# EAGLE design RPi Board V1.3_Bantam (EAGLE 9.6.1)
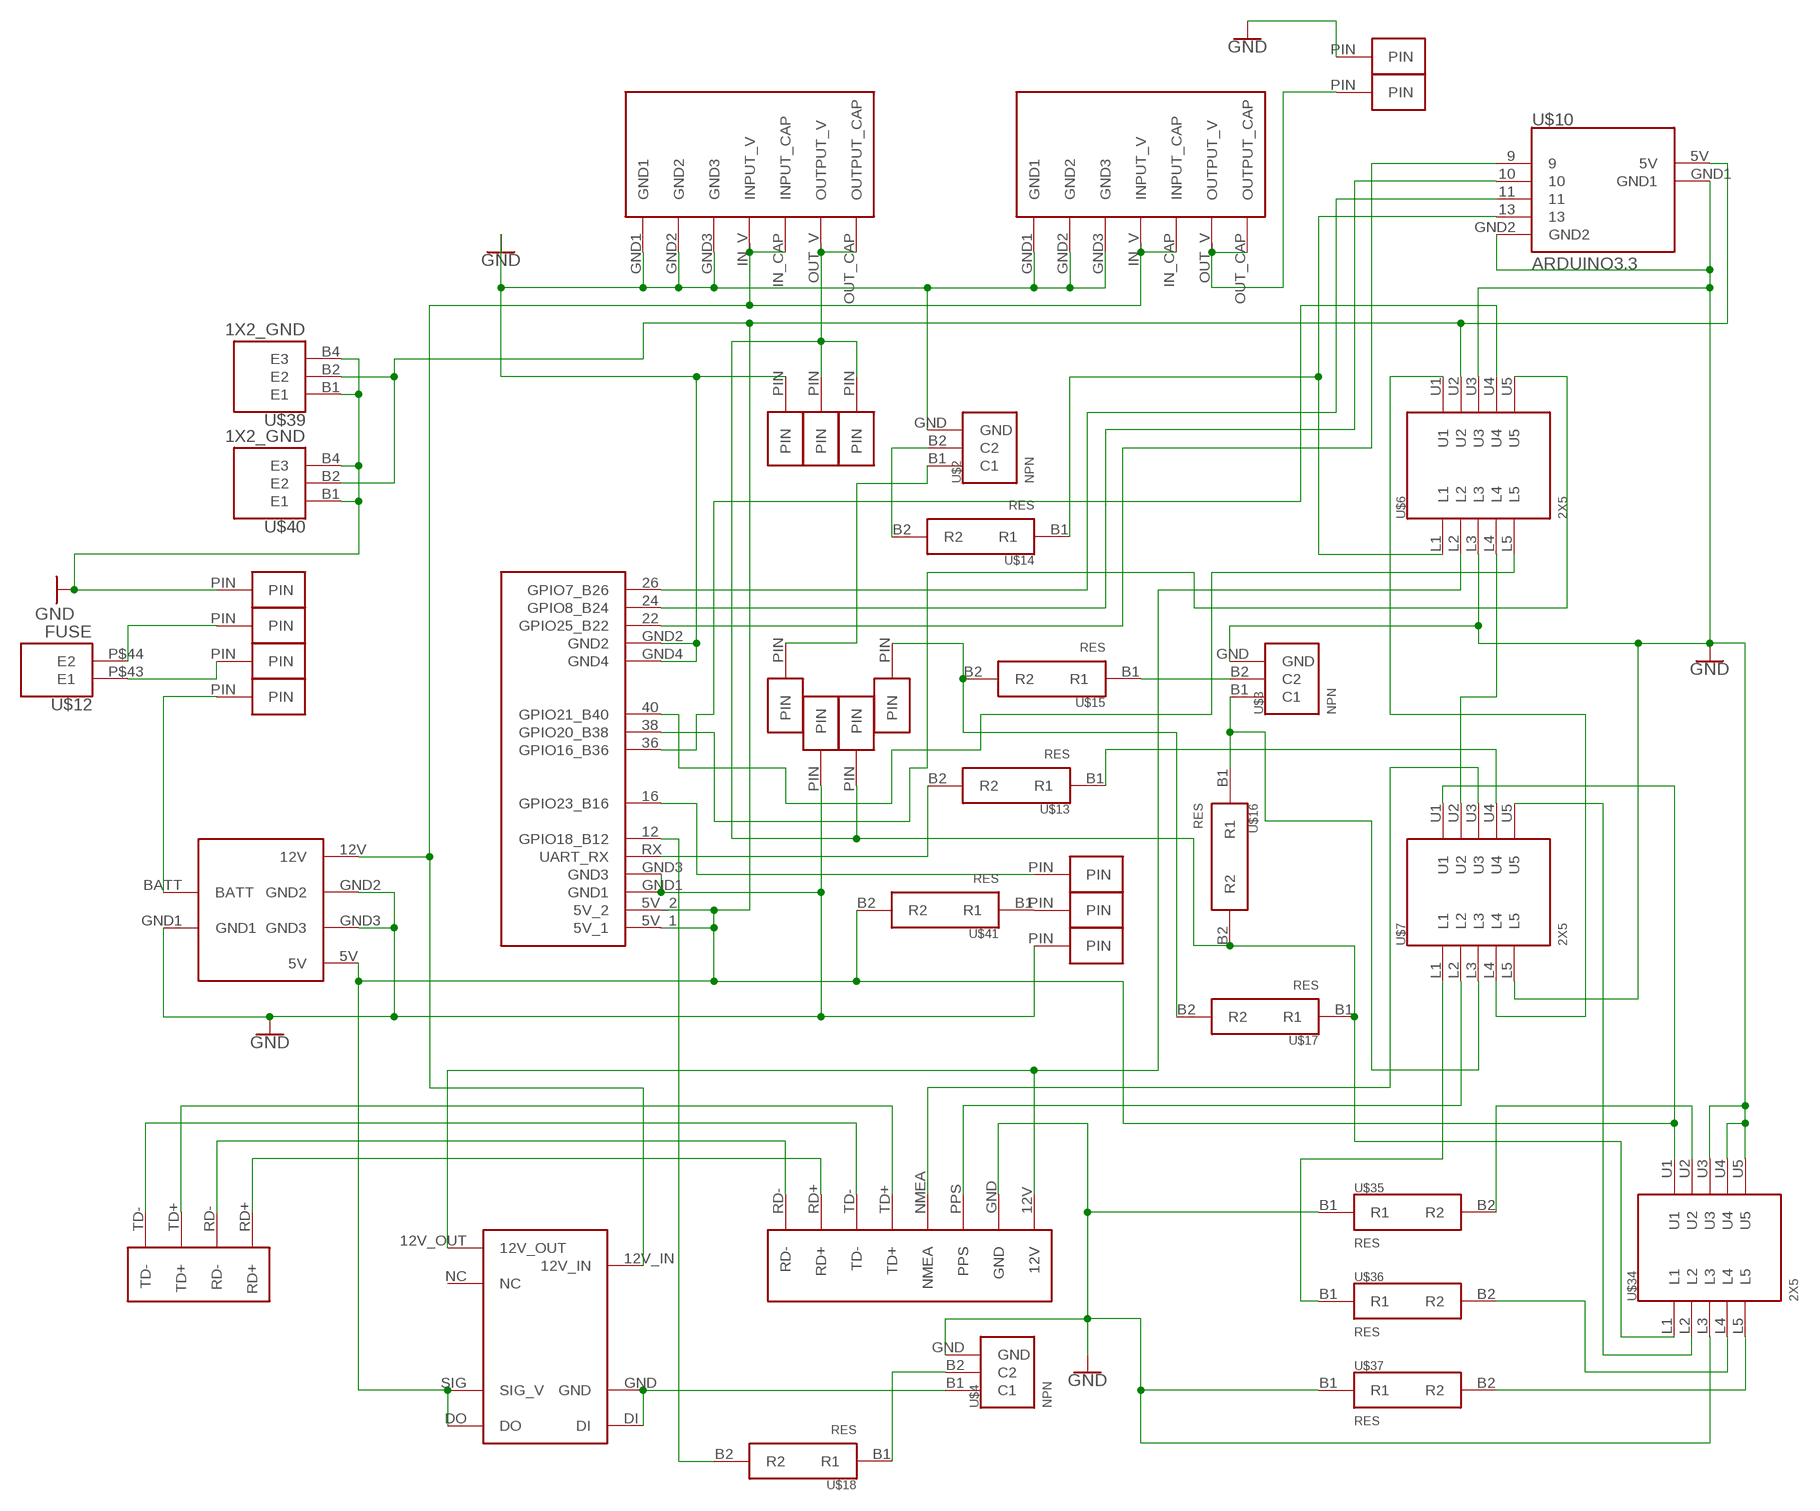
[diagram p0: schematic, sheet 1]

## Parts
U$1  RPI_1X20  [F_RPI_1X20]
U$2  NPN  [F_NPN]
U$3  NPN  [F_NPN]
U$4  NPN  [F_NPN]
U$5  LIDAR  [F_LIDAR]
U$6  2X5  [F_2X5]
U$7  2X5  [F_2X5]
U$8  3.3V_REG  [F_3.3V_REG]
U$9  9V_REG  [F_9V_REG]
U$10  ARDUINO3.3  [F_ARDUINO3.3]
U$11  ETH  [F_ETH]
U$12  FUSE  [F_FUSE]
U$13  RES  [F_RES]
U$14  RES  [F_RES]
U$15  RES  [F_RES]
U$16  RES  [F_RES]
U$17  RES  [F_RES]
U$18  RES  [F_RES]
U$19  1X1  [F_1X1]
U$20  1X1  [F_1X1]
U$21  1X1  [F_1X1]
U$22  1X1  [F_1X1]
U$23  12V_5V_REG  [F_12V_5V_REG]
U$24  1X1  [F_1X1]
U$25  RELAY  [F_RELAY]
U$26  1X1  [F_1X1]
U$27  1X1  [F_1X1]
U$28  1X1  [F_1X1]
U$29  1X1  [F_1X1]
U$30  1X1  [F_1X1]
U$31  1X1  [F_1X1]
U$32  1X1  [F_1X1]
U$33  1X1  [F_1X1]
U$34  2X5  [F_2X5]
U$35  RES  [F_RES]
U$36  RES  [F_RES]
U$37  RES  [F_RES]
U$38  1X1  [F_1X1]
U$39  1X2_GND  [F_1X2_GND]
U$40  1X2_GND  [F_1X2_GND]
U$41  RES  [F_RES]
U$42  1X1  [F_1X1]
U$43  1X1  [F_1X1]

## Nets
GND: U$1.GND1 U$1.GND2 U$1.GND3 U$1.GND4 U$2.GND U$3.GND U$4.GND U$5.GND U$6.L3 U$6.U3 U$7.L5 U$8.GND1 U$8.GND2 U$8.GND3 U$9.GND1 U$9.GND2 U$9.GND3 U$10.GND1 U$10.GND2 U$22.PIN U$23.GND1 U$23.GND2 U$23.GND3 U$26.PIN U$28.PIN U$30.PIN U$34.L3 U$34.U3 U$34.U4 U$34.U5 U$35.B1(R1) U$37.B1(R1) U$39.B1(E1) U$39.B4(E3) U$40.B1(E1) U$40.B4(E3) U$43.PIN
N$1: U$12.P$44(E2) U$19.PIN
N$2: U$12.P$43(E1) U$20.PIN
N$3: U$21.PIN U$23.BATT
N$4: U$5.RD- U$11.RD-
N$5: U$5.RD+ U$11.RD+
N$6: U$5.TD- U$11.TD-
N$7: U$41.B1(R1) U$42.PIN
N$8: U$8.OUT_CAP(OUTPUT_CAP) U$8.OUT_V(OUTPUT_V) U$16.B2(R2) U$17.B1(R1) U$24.PIN U$27.PIN U$32.PIN U$34.L1
N$9: U$5.TD+ U$11.TD+
N$10: U$5.PPS U$7.L2
N$11: U$7.U4 U$13.B1(R1)
N$12: U$1.RX(UART_RX) U$13.B2(R2)
N$13: U$5.12V U$6.L2 U$25.12V_OUT
N$14: U$6.U1 U$7.L4
N$15: U$6.L4 U$7.U2
N$16: U$1.5V_1 U$1.5V_2 U$6.U2 U$7.U1 U$10.5V U$23.5V U$25.DO U$25.SIG(SIG_V) U$34.U1 U$39.B2(E2) U$40.B2(E2) U$41.B2(R2)
N$17: U$5.NMEA U$7.U3
N$19: U$1.22(GPIO25_B22) U$10.9
N$20: U$1.24(GPIO8_B24) U$10.10
N$21: U$8.IN_CAP(INPUT_CAP) U$8.IN_V(INPUT_V) U$9.IN_CAP(INPUT_CAP) U$9.IN_V(INPUT_V) U$23.12V U$25.12V_IN
N$22: U$1.26(GPIO7_B26) U$10.11
N$23: U$9.OUT_CAP(OUTPUT_CAP) U$9.OUT_V(OUTPUT_V) U$29.PIN
N$24: U$2.B2(C2) U$14.B2(R2)
N$25: U$6.L1 U$10.13 U$14.B1(R1)
N$26: U$2.B1(C1) U$31.PIN
N$27: U$15.B2(R2) U$17.B2(R2) U$33.PIN
N$28: U$3.B2(C2) U$15.B1(R1)
N$29: U$3.B1(C1) U$7.L3 U$16.B1(R1)
N$30: U$4.B1(C1) U$25.DI U$25.GND
N$31: U$4.B2(C2) U$18.B1(R1)
N$32: U$1.38(GPIO20_B38) U$6.U5
N$33: U$1.12(GPIO18_B12) U$18.B2(R2)
N$34: U$1.36(GPIO16_B36) U$6.U4
N$35: U$7.U5 U$34.L2
N$36: U$34.U2 U$35.B2(R2)
N$37: U$1.16(GPIO23_B16) U$38.PIN
N$38: U$34.L5 U$37.B2(R2)
N$39: U$34.L4 U$36.B2(R2)
N$40: U$7.L1 U$36.B1(R1)
N$42: U$1.40(GPIO21_B40) U$6.L5
Unconnected: U$25.NC

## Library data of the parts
U$1 = OpenMMS_Bantam:RPI_1X20
U$2-U$4 = OpenMMS_Bantam:NPN
U$5 = OpenMMS_Bantam:LIDAR
U$6 U$7 U$34 = OpenMMS_Bantam:2X5
U$8 = OpenMMS_Bantam:3.3V_REG
U$9 = OpenMMS_Bantam:9V_REG
U$10 = OpenMMS_Bantam:ARDUINO3.3
U$11 = OpenMMS_Bantam:ETH
U$12 = OpenMMS_Bantam:FUSE
U$13-U$18 U$35-U$37 U$41 = OpenMMS_Bantam:RES
U$19-U$22 U$24 U$26-U$33 U$38 U$42 U$43 = OpenMMS_Bantam:1X1
U$23 = OpenMMS_Bantam:12V_5V_REG
U$25 = OpenMMS_Bantam:RELAY
U$39 U$40 = OpenMMS_Bantam:1X2_GND

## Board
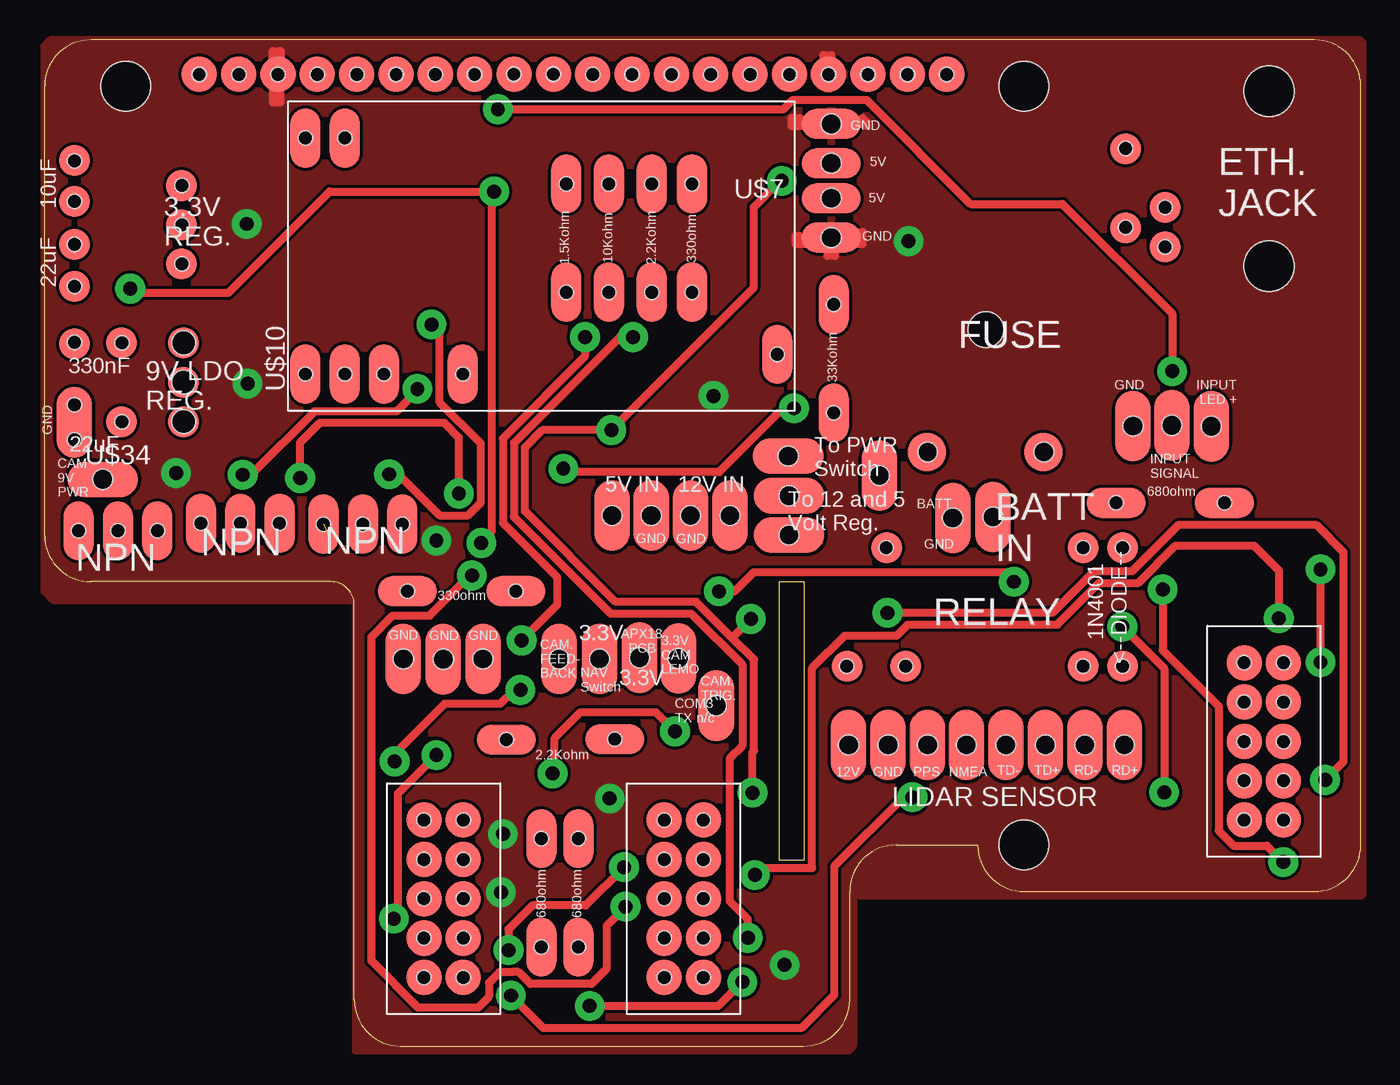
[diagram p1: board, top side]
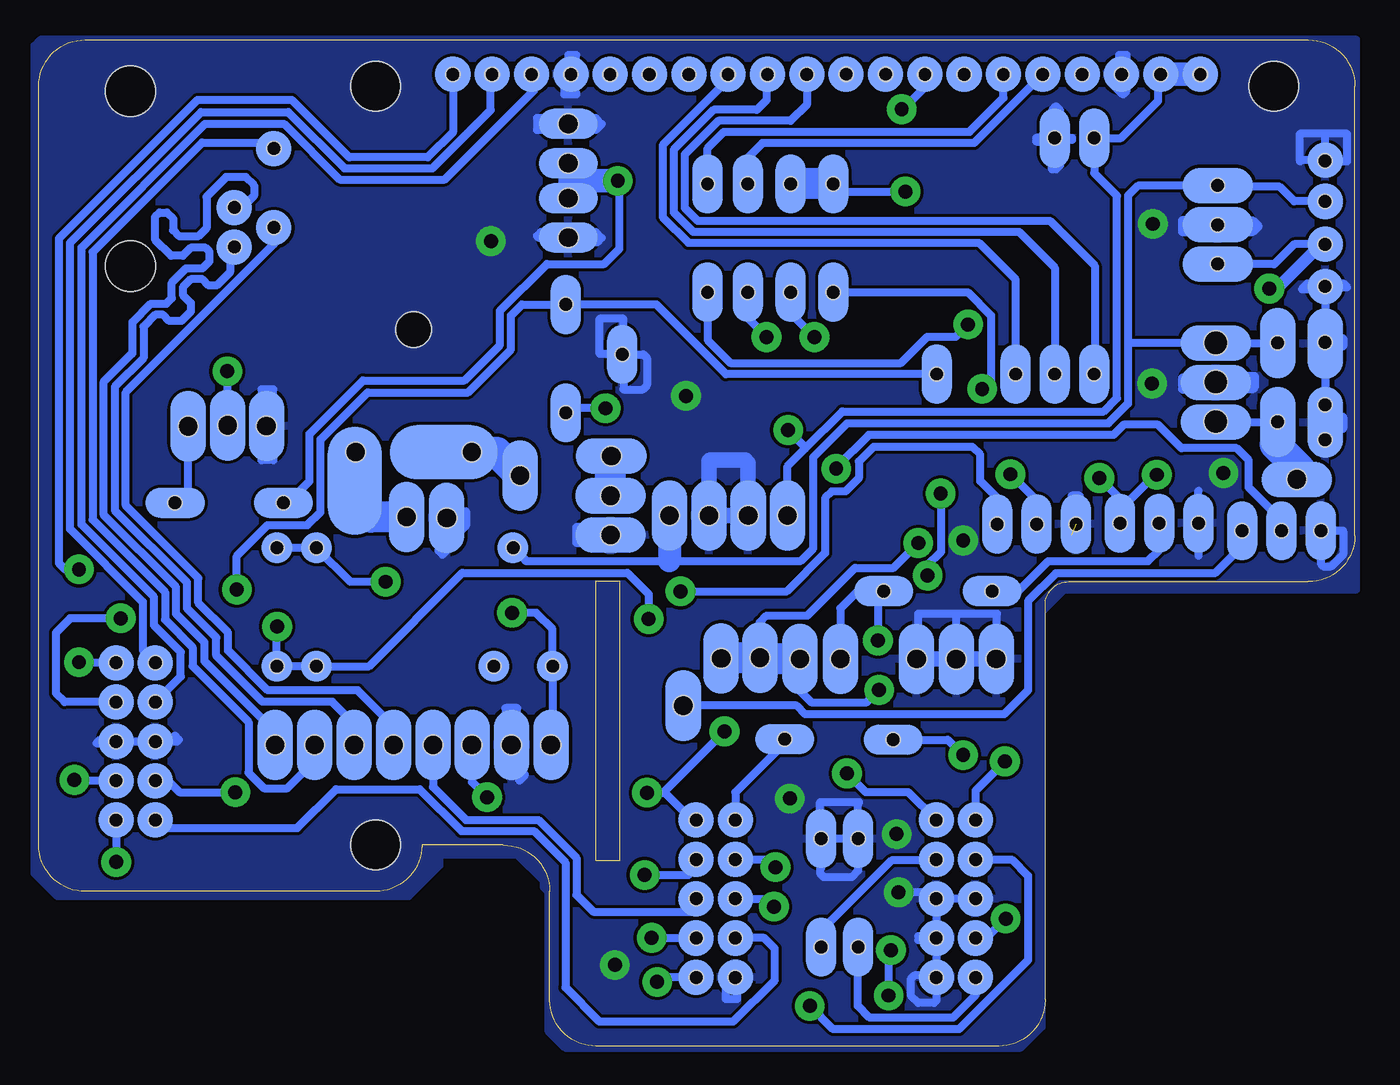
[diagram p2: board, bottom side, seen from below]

Size 85 x 65 mm. Coordinates in mm from the lower left corner, seen from the top.
Outline: 49.05,12 47.45,12 47.45,30 49.05,30 49.05,12
Outline: 20,3 arc90 23,0 49,0 arc90 52,3 52,10 arc-90 55,13 60.25,13 arc90 63.25,10 82,10 arc90 85,13 85,62 arc90 82,65 3,65 arc90 0,62 0,33 arc90 3,30 18.5,30 arc-90 20,28.5 20,3
Copper layers (1*16): Top 0.035mm / dielectric 1.5mm / Bottom 0.035mm
Design rules "OpenMMS_Bantam": minimum track width 20mil, minimum drill 0.9mm, track to track 8mil, track to pad 8mil, pad to pad 8mil, via to via 8mil, smd to smd 8mil, copper to edge 0mil, drill to drill 0mil, minimum pad ring 20mil, minimum via ring 20mil, stop-mask expansion 4mil, vias tented up to drill 0mil, thermal gap 8mil
Holes 3.2 mm at 5.25,62 63.25,62 63.25,13
Holes 0.9 mm at 9.98,62.76 12.55,62.76 15.06,62.76 17.63,62.76 20.17,62.76 22.71,62.76 25.25,62.76 27.76,62.76 30.3,62.79 32.84,62.79 35.41,62.76 37.95,62.76 40.49,62.76 43.03,62.76 45.57,62.76 48.11,62.76 50.62,62.76 53.16,62.76 55.73,62.76 58.27,62.76

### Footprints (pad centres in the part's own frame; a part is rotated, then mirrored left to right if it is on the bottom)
F_RPI_1X20 = smd 2.3 x 2.3 bottom: 5V_1 0,0; 5V_2 2.54,0; 12 12.7,0; 16 17.78,0; 22 25.4,0; 24 27.94,0; 26 30.48,0; 36 43.18,0; 38 45.72,0; 40 48.26,0; GND1 5.08,0; GND2 40.64,0; P$21 7.62,0; P$22 15.24,0; P$23 20.32,0; P$24 22.86,0; P$25 33.02,0; P$26 35.56,0; P$27 38.1,0; RX 10.16,0 | smd 2.3 x 2.3: GND3 5.08,0; GND4 40.64,0; P$1 0,0; P$2 2.54,0; P$4 10.16,0; P$5 12.7,0; P$6 17.78,0; P$7 25.4,0; P$8 27.94,0; P$9 30.48,0; P$11 43.18,0; P$12 45.72,0; P$13 48.26,0; P$14 7.62,0; P$15 15.24,0; P$16 20.32,0; P$17 22.86,0; P$18 33.02,0; P$19 35.56,0; P$20 38.1,0 | hole 0.9: 0,0; 2.54,0; 5.08,0; 7.62,0; 10.16,0; 12.7,0; 15.24,0; 17.78,0; 20.32,0; 22.86,0; 25.4,0; 27.94,0; 30.48,0; 33.02,0; 35.56,0; 38.1,0; 40.64,0; 43.18,0; 45.72,0; 48.26,0
F_NPN = smd 1.93 x 3.81 bottom: B1 -2.54,0; B2 0,0; GND 2.54,0 | smd 1.93 x 3.81: B4 -2.54,0; B5 0,0; B6 2.54,0 | hole 0.9: -2.54,0; 0,0; 2.54,0
F_LIDAR = smd 2.299 x 4.572 bottom: 12V -9.04,-0.23; GND -6.49,-0.23; NMEA -1.429,-0.23; PPS -3.94,-0.23; RD+ 8.76,-0.23; RD- 6.21,-0.23; TD+ 3.66,-0.23; TD- 1.11,-0.23 | smd 2.299 x 4.572: P$237 -9.04,-0.23; P$238 -6.49,-0.23; P$239 -3.94,-0.23; P$240 -1.429,-0.23; P$241 1.11,-0.23; P$242 3.66,-0.23; P$243 6.21,-0.23; P$244 8.76,-0.23 | hole 1.27: -9.03,-0.22; -6.48,-0.22; -3.93,-0.22; -1.43,-0.22; 1.12,-0.22; 3.67,-0.22; 6.22,-0.22; 8.77,-0.22
F_2X5 = smd 2.286 x 2.286: B1 -5.08,-1.27; B2 -2.54,-1.27; B3 0,-1.27; B4 2.54,-1.27; B5 5.08,-1.27; B6 5.08,1.27; B7 2.54,1.27; B8 0,1.27; B9 -2.54,1.27; B20 -5.08,1.27 | smd 2.286 x 2.286 bottom: L1 -5.08,-1.27; L2 -2.54,-1.27; L3 0,-1.27; L4 2.54,-1.27; L5 5.08,-1.27; U1 -5.08,1.27; U2 -2.54,1.27; U3 0,1.27; U4 2.54,1.27; U5 5.08,1.27 | hole 0.9: -5.08,-1.27; -2.54,-1.27; 0,-1.27; 2.54,-1.27; 5.08,-1.27; 5.08,1.27; 2.54,1.27; 0,1.27; -2.54,1.27; -5.08,1.27
F_3.3V_REG = smd 4.572 x 2.299 bottom: GND1 3.133,-0.647; IN_V 3.133,1.883; OUT_V 3.133,-3.177 | smd 2.299 x 2.299 bottom: GND2 -3.798,3.515; GND3 -3.798,-4.623; IN_CAP -3.788,0.867; OUT_CAP -3.788,-1.907 | smd 2 x 2: P$201 3.133,-3.177; P$202 3.133,-0.647; P$203 3.133,1.883; P$204 -3.788,-1.907; P$205 -3.798,3.515; P$206 -3.788,0.867; P$207 -3.798,-4.623 | hole 0.9: -3.788,3.475; -3.788,-4.613; -3.778,0.877; -3.778,-1.897; 3.143,-3.167; 3.143,-0.637; 3.143,1.893
F_9V_REG = smd 4.572 x 2.299 bottom: GND1 3.26,-0.52; IN_V 3.26,2.03; OUT_V 3.26,-3.07 | smd 2.299 x 4.572 bottom: GND2 -3.798,1.991; GND3 -3.798,-3.099; IN_CAP -0.74,2.03; OUT_CAP -0.74,-3.07 | smd 2 x 2: P$201 3.26,2.03; P$202 3.26,-0.52; P$203 3.26,-3.07; P$204 -0.74,2.03; P$205 -3.798,1.991; P$206 -0.74,-3.07 | smd 2.299 x 4.572: P$207 -3.798,-3.099 | hole 0.9: -3.788,2.078; -3.788,-1.946; -0.73,-3.06; -0.73,2.04; -3.788,-4.232 | hole 1.524: 3.27,2.04; 3.27,-0.5; 3.27,-3.04
F_ARDUINO3.3 = smd 3.81 x 1.93 bottom: 5V 7.62,13.97; 9 -7.62,13.97; 10 -7.62,11.43; 11 -7.62,8.89; 13 -7.62,3.81; GND1 7.62,11.43; GND2 -6.35,-16.51 | smd 3.81 x 1.93: B4 -7.62,13.97; B6 -7.62,11.43; B7 -7.62,8.89; B8 -7.62,3.81; B9 -6.35,-16.51; B10 7.62,11.43; B11 7.62,13.97 | hole 0.9: -7.62,13.97; -7.62,11.43; -7.62,8.89; -7.62,3.81; -6.35,-16.51; 7.62,11.43; 7.62,13.97
F_ETH = smd 2 x 2: P$222 -5.79,2.08; P$223 -3.24,-1.72; P$224 -5.79,-3.02; P$225 -3.24,-4.27 | smd 2.3 x 2.3 bottom: RD+ -3.24,-1.72; RD- -5.79,2.08; TD+ -3.24,-4.27; TD- -5.79,-3.02 | hole 3.25: 3.47,5.79; 3.47,-5.51 | hole 0.9: -5.78,2.09; -5.78,-3.01; -3.23,-1.71; -3.23,-4.26
F_FUSE = smd 3.5 x 7 bottom: P$43 -0.44,2.05 | smd 7 x 3.5 bottom: P$44 -2.29,-3.7 | smd 2.5 x 2.5: P$175 -0.44,3.9; P$176 -0.44,-3.6 | hole 2.3: 7.47,0.11 | hole 1.25: -0.43,3.86; -0.43,-3.64
F_RES = smd 1.93 x 3.81 bottom: B1 0,3.5; B2 0,-3.5 | smd 1.93 x 3.81: T1 0,3.5; T2 0,-3.5 | hole 0.9: 0,3.5; 0,-3.5
F_1X1 = smd 4.572 x 2.299: P$1 0,0 | smd 4.572 x 2.299 bottom: PIN 0,0 | hole 1.27: 0,0
F_12V_5V_REG = smd 2.299 x 4.572 bottom: 5V 6.35,0; 12V -1.27,0; GND2 1.27,0; GND3 3.81,0 | smd 4.572 x 2.299 bottom: BATT -5.08,-1.27; GND1 -5.08,1.27 | smd 4.572 x 2.299: P$1 -5.08,1.27; P$2 -5.08,-1.27 | smd 2.299 x 4.572: P$3 -1.27,0; P$4 1.27,0; P$5 3.81,0; P$6 6.35,0 | hole 1.27: -5.08,1.27; -5.08,-1.27; -1.27,0; 1.27,0; 3.81,0; 6.35,0
F_RELAY = smd 2 x 2 bottom: 12V_IN 3.88,6.39; 12V_OUT -3.77,8.94; DI 3.88,-8.86; DO -3.77,-8.86; GND 3.88,-6.31; NC -3.77,5.14; SIG -3.77,-6.31 | smd 2 x 2: P$185 -3.77,8.94; P$186 3.88,6.39; P$187 -3.77,5.14; P$188 -3.77,-6.31; P$189 3.88,-6.31; P$190 -3.77,-8.86; P$191 3.88,-8.86 | hole 0.9: -3.76,8.95; -3.76,5.15; 3.89,6.4; -3.76,-6.3; -3.76,-8.85; 3.89,-6.3; 3.89,-8.85
F_1X2_GND = smd 3.81 x 1.93 bottom: B1 0,1.27; B2 0,-1.27 | smd 3.81 x 1.93: B4 0,1.27; B5 0,-1.27 | hole 1.27: 0,1.27; 0,-1.27

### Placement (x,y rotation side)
U$1  9.99,62.77 0 top
U$2  4.74,33.3 180 top
U$3  12.64,33.78 180 top
U$4  20.56,33.73 180 top
U$5  60.96,19.68 0 top
U$6  78.74,19.68 90 top
U$7  41.27,9.53 270 top
U$8  5.72,53.7 0 top
U$9  5.72,43.39 0 top
U$10  30.81,51.03 90 top
U$11  75.61,55.88 0 top
U$12  60.89,38.81 90 top
U$13  39.21,52.2 180 top
U$14  50.97,44.4 0 top
U$15  26.93,29.4 90 top
U$16  33.69,52.2 180 top
U$17  36.45,52.2 0 top
U$18  41.81,52.2 180 top
U$19  61.24,34.18 90 top
U$20  53.92,36.87 270 top
U$21  48.03,38.12 0 top
U$22  58.65,34.12 90 top
U$23  42.99,34.28 180 top
U$24  40.93,25.05 270 top
U$25  60.76,28.31 90 top
U$26  23.16,25.02 90 top
U$27  38.42,25.09 90 top
U$28  25.74,24.99 90 top
U$29  3.75,36.61 180 top
U$30  28.3,25.02 90 top
U$31  43.37,21.99 90 top
U$32  35.84,25.02 90 top
U$33  33.22,25.02 90 top
U$34  25.77,9.53 270 top
U$35  34.47,9.9 0 top
U$36  33.33,19.82 270.3 top
U$37  32.09,9.9 0 top
U$38  72.8,40.1 90 top
U$39  50.8,58.3 0 top
U$40  50.8,53.5 180 top
U$41  72.69,35.09 270 top
U$42  75.34,40.03 90 top
U$43  70.29,40.06 90 top

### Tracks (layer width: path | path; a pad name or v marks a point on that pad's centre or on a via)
GND  (via drill 0.9)  (1 unrouted)
  Top 0.508: U$1.GND3 15.07,62.32 14.73,61.98 14.73,60.96 15.24,60.96 15.24,61.94 15.78,62.48 15.78,63.06 15.37,63.48 15.07,63.48 | 15.07,63.48 15.01,63.48 14.73,63.75 14.73,64.26 15.24,64.26 15.24,63.64 15.07,63.48 | U$1.GND4 50.29,63.11 50.29,64.01 50.8,64.01 50.8,63.64 50.63,63.48 | U$39.B1 49.91,59.57 | 49.91,59.57 49.14,59.57 48.77,59.94 48.26,59.94 48.26,59.44 49.78,59.44 49.91,59.57 | U$39.B1 52.46,59.57 52.83,59.94 53.09,59.69 53.09,59.44 52.95,59.57 U$39.B1 | U$40.B1 49.91,52.23 | 49.91,52.23 48.86,52.23 48.77,52.32 48.51,52.32 48.51,51.82 49.5,51.82 49.91,52.23 | U$40.B1 51.15,52.58 52.83,52.58 52.83,51.82 52.07,51.82 51.69,52.2 | 51.69,52.2 51.69,52.32 | U$40.B1 51.66,52.23 51.69,52.2 | U$40.B1 50.55,51.98 50.55,51.05 51.05,51.05 51.05,51.98 U$40.B1
  Bottom 0.508: 25.71,25.02 U$28.PIN | U$28.PIN 25.77,25.02 | U$10.GND1 18.68,58.65 | 18.68,58.65 18.31,58.65 18.29,58.67 18.26,58.65 18.26,58.55 18.57,58.55 18.68,58.65 | 19.09,57.95 18.68,58.36 18.68,58.65 | 19.09,59.35 19.3,59.57 | 19.3,59.57 19.56,59.82 19.56,60.45 19.3,60.71 19.05,60.45 19.3,60.2 19.3,59.57 | 18.68,58.65 18.68,58.94 19.09,59.35 | 19.09,59.35 19.67,59.35 20.35,58.67 20.57,58.67 20.57,58.42 20.15,58.42 19.67,57.95 19.09,57.95 | 19.05,57.98 19.05,56.9 19.3,56.64 19.56,56.64 19.56,57.48 19.09,57.95 | U$1.GND4 50.29,63.11 50.29,64.01 50.8,64.01 50.8,63.64 50.63,63.48 50.93,63.48 51.34,63.06 51.34,62.48 51.05,62.2 | 51.05,62.2 50.92,62.06 50.8,62.06 50.29,61.55 50.29,61.47 51.05,61.47 51.05,62.2 | U$39.B1 49.91,59.57 | 49.91,59.57 49.4,59.57 49.02,59.94 48.64,59.56 49.02,59.18 49.52,59.18 49.91,59.57 | U$39.B1 51.17,59.94 52.07,59.94 | 52.07,59.94 52.83,59.94 52.83,59.18 52.07,59.18 | U$39.B1 51.7,59.57 52.07,59.94 | 52.23,52.23 U$40.B1 49.91,52.23 | 52.23,52.23 52.58,52.58 52.83,52.32 52.74,52.23 52.23,52.23 | 49.91,52.23 49.37,52.23 49.02,52.58 48.64,52.2 48.9,51.94 49.62,51.94 49.91,52.23 | U$10.GND2 47.24,44.76 47.24,46.99 48.77,46.99 48.77,44.7 47.34,44.7 U$10.GND2 | U$10.GND2 45.95,44.68 45.72,44.45 45.72,42.67 45.97,42.42 47.24,42.42 47.24,44.6 U$10.GND2 | U$8.GND2 1.86,57.15 0.51,57.15 0.51,58.93 2.03,58.93 | 2.03,58.93 3.56,58.93 3.56,57.15 3.5,57.21 U$8.GND2 | U$8.GND2 1.92,58.81 2.03,58.93 | U$8.GND3 U$9.GND2 | U$8.GND3 0.96,49.07 0.76,49.28 0.51,49.02 0.99,49.02 1.64,48.38 2.22,48.38 2.74,48.9 3.43,48.9 3.05,49.28 2.85,49.07 U$8.GND3 | U$9.GND2 1.58,45.72 0.76,45.72 0.76,45.21 1.19,45.21 1.64,44.76 2.22,44.76 2.67,45.21
  Bottom 0.508: U$9.GND2 2.26,45.72 | U$9.GND2 U$9.GND3 | U$9.GND3 2.02,40.39 | 2.33,39.88 U$9.GND3 | U$9.GND3 1.57,40.64 0.76,40.64 0.76,39.88 1.51,39.88 U$9.GND3 | 8.27,42.16 8.02,42.42 6.6,42.42 6.48,42.55 6.48,43.31 8.54,43.31 U$9.GND1 9.29,43.18 11.18,43.18 11.18,42.42 9.96,42.42 | U$3.GND 10.1,35.87 | U$3.GND 10.1,33.08 | 10.1,33.08 10.1,31.69 | U$3.GND | U$3.GND 9.4,33.78 | 9.4,33.78 9.39,33.78 | 9.4,33.78 9.4,33.49 9.81,33.08 10.1,33.08 | 18.31,33.02 17.73,33.02 | U$26.PIN 23.11,25.07 23.11,27.94 25.65,27.94 | 25.65,27.94 28.19,27.94 28.19,25.13 U$30.PIN | U$28.PIN 25.75,27.85 25.65,27.94 | 39.18,37.66 39.37,37.85 | 41.72,37.78 41.66,37.85 | U$23.GND1 48.59,33.53 50.29,33.53 50.29,32.51 48.83,32.51 48.44,32.12 47.7,32.12 47.18,32.64 47.18,33.01 | 57.76,34.12 57.76,33.27 | 57.76,33.27 57.4,33.63 57.4,34.54 57.83,34.12 U$22.PIN 59.18,33.58 59.18,32 58.93,31.75 57.76,32.92 57.76,33.27 | U$37.B1 U$35.B1 | U$35.B1 34.54,13.47 34.54,15.75 32,15.75 32.09,15.66 U$37.B1 | U$37.B1 32.09,11.34 32.51,10.92 34.29,10.92 34.54,11.18 34.54,11.43 34.47,11.5 U$35.B1 | U$34.L3 U$34.U3 | U$34.U3 U$34.U4 | U$34.U4 U$34.U5 | U$34.U5 27.17,4.57 28.45,4.57 28.7,4.32 28.7,3.86 28.7,3.3 28.19,2.79 27.18,2.79 27.04,2.93 U$34.U5 | U$34.U3 27.45,9.94 v29.47,9.94 | U$34.U4 27.17,7.11 28.19,7.11 28.19,6.86 27.91,6.86 27.33,6.28 26.75,6.28 26.34,6.69 26.34,6.99 | 39.5,4.45 U$7.L5 40.64,3.81 40.64,3.05 39.88,3.05 39.88,3.58 39.3,4.15 39.3,4.45 | 79.31,19.68 U$6.L3 80.14,19.81 81.03,19.81 81.28,19.56 80.88,19.56 80.3,18.98 79.72,18.98 79.31,19.39 79.31,19.68 | 79.31,19.68 U$6.U3 76.58,19.68 | 76.58,19.68 76.2,20.07 75.95,19.81 76.07,19.68 76.58,19.68
  Bottom 0.508: U$1.GND3 14.73,63.11 14.73,64.01 15.24,64.01 15.24,63.64 15.07,63.48 15.37,63.48 15.78,63.06 15.78,62.26 14.99,61.47 14.73,61.72 15.07,62.06 U$1.GND3 | U$8.GND1 6.89,53.05 6.6,53.34 6.22,52.96 6.6,52.58 8.35,52.58 8.57,52.35 9.15,52.35 9.38,52.58 11.18,52.58 11.18,53.34 9.14,53.34 U$8.GND1 | U$2.GND 0.78,33.3 0.76,33.27 0.76,31.75 1.52,30.99 2.03,30.99 2.2,31.16 U$2.GND | 17.78,34.48 17.78,35.56 18.29,35.56 18.29,34.99 17.78,34.48 | U$5.GND 54.1,19.82 54.1,21.84 54.86,21.84 54.86,21.11 53.59,19.83 53.59,19.1 53.98,18.71 53.98,17.14 53.59,17.53 54.47,18.4 U$5.GND | U$43.PIN 69.85,40.5 69.85,42.42 70.61,42.42 70.61,41.64 69.4,40.43 69.4,39.69 70.61,38.48 70.61,37.85 69.85,37.85 69.85,38.1 70.29,38.54 U$43.PIN
  Bottom 1: U$26.PIN 25.71,25.02 | 25.77,25.02 U$30.PIN | 39.18,37.66 U$23.GND3 U$23.GND2 41.72,37.78 | 41.66,37.85 39.37,37.85
  other vias: 55.8,52 43.2,42 8.49,37.02 25.3,32.67 36.49,15.99 47.79,5.25 29.6,13.7 13.06,53.11 13.11,42.8
  pour Bottom: -0.1,65 84.9,65 85.3,64.6 85.3,11.2 83.8,9.7 61.1,9.7 59.1,11.7 59.1,12.5 59,12.4 54.1,12.4 52.4,10.7 52.4,10.3 52.1,10 52.1,1 51,-0.1 21.6,-0.1 20.22,1.28 20.22,28.08 18.8,29.5 -0.1,29.5
  pour Top: 0.4,65 84.9,65 85.1,64.8 85.1,9.8 85,9.7 52.7,9.7 52.2,10.2 52.2,0 51.9,-0.3 20.11,-0.3 20.11,28.8 0.6,28.8 0,29.4 0,64.6
N$1
  Bottom 0.508: U$12.P$44 64.59,35.22 63.55,34.18
  Bottom 2: U$19.PIN 63.55,34.18
N$2
  Bottom 2: U$12.P$43 55.42,38.37 U$20.PIN
N$3
  Bottom 0.508: 48.07,38.12 U$21.PIN
  Bottom 2: U$23.BATT 48.07,38.12
N$4
  Bottom 0.508: U$11.RD- 70.22,58.37 74.45,58.37 81.52,51.3 81.52,34 76.85,29.33 76.85,27.55 75.06,25.77 75.06,24.54 71.46,20.94 71.46,17.66 70.45,16.65 68.95,16.65 67.17,18.43 U$5.RD-
N$5
  Bottom 0.508: U$5.RD+ 69.72,20.29 74.3,24.86 74.3,26.08 76.13,27.92 76.13,29.65 80.79,34.31 80.79,42.94 79.03,44.7 78.98,44.7 78.94,44.74 78.94,46.78 77.77,47.95 76.76,47.95 76.4,48.31 76.4,49.32 75.48,50.24 74.42,50.24 73.97,50.69 73.97,51.31 74.23,51.56 75.18,51.56 75.69,51.05 76.45,51.05 77.47,52.07 77.47,53.59 77.22,53.85 76.71,53.85 76.33,53.47 76.33,52.7 75.95,52.32 74.68,52.32 74.17,52.83 74.17,54.86 72.9,56.13 71.63,56.13 71.09,55.6 71.09,54.92 71.86,54.16 U$11.RD+
N$6
  Bottom 0.508: U$5.TD- 62.07,20.65 64.4,22.98 70.2,22.98 72.77,25.55 72.77,26.71 74.69,28.63 74.69,30.23 79.37,34.91 79.37,42.23 69.81,51.79 U$11.TD-
N$7
  Bottom 0.508: U$41.B1 75.34,35.94 U$42.PIN
N$8  (via drill 0.9)
  Top 0.508: v5.53,48.93 5.81,48.65 11.86,48.65 18.41,55.2 v29.03,55.2 28.89,55.06 28.89,33.29 28.2,32.6 v28.2,32.5 | v30.73,23.01 30.58,22.86 30.18,22.86 29.43,22.11 25.83,22.11 22.6,18.88 v22.6,18.4
  Bottom 0.508: v29.03,55.2 33.19,55.2 U$16.B2 | v28.2,32.5 29.8,30.9 32.28,30.9 35.37,27.81 37.99,27.81 38.42,27.38 U$27.PIN 38.35,25.02 | v30.73,23.01 31.53,22.21 35.11,22.21 35.84,22.95 U$32.PIN | v22.6,18.4 24.5,16.5 U$34.L1 | 40.89,25.09 U$24.PIN | U$8.OUT_V 8.83,50.5 5.22,50.5 3.93,51.79 U$8.OUT_CAP 2.18,51.79 | 5.04,48.93 v5.53,48.93
  Bottom 0.8: 5.04,48.93 2.18,51.79
  Bottom 2: U$16.B2 U$17.B1 | U$32.PIN 38.35,25.02 | U$27.PIN 40.89,25.09
N$9
  Bottom 0.508: U$5.TD+ 64.62,20.82 66.05,22.25 70.55,22.25 73.53,25.23 73.53,26.4 75.42,28.29 75.42,29.95 80.08,34.61 80.08,42.6 78.23,44.45 78.23,46.48 77.47,47.24 76.96,47.24 76.56,46.84 75.8,46.84 75.18,47.45 75.18,48.01 75.69,48.51 75.69,49.02 75.18,49.53 74.42,49.53 74.02,49.13 73.51,49.13 72.64,49.99 72.64,51.33 U$11.TD+
N$10  (via drill 0.9)
  Top 0.508: v37.42,11.56 34.95,9.09 31.5,9.09 29.96,7.55 v29.96,6.2 | v30.12,3.27 32.22,1.17 48.87,1.17 50.99,3.29 50.99,11.61 55.46,16.08 v56.04,16.08
  Bottom 0.508: U$7.L2 37.92,12.06 v37.42,11.56 | v29.96,6.2 30.12,6.05 v30.12,3.27 | U$5.PPS 57.02,17.05 v56.04,16.08
N$11  (via drill 0.9)
  Top 0.508: v38,45.8 37.15,45.8 30.31,38.97 30.31,34.19 36.56,27.94 41.76,27.94 45.06,24.65 45.06,19.4 44.24,18.58 44.24,9.38 45.42,8.21 v45.42,7
  Bottom 0.508: U$13.B1 39.21,47.01 v38,45.8 | v45.42,7 45.4,6.99 U$7.U4
N$12
  Bottom 0.508: U$1.RX 24.6,58.33 38.27,58.33 39.21,57.39 U$13.B2
N$13  (via drill 0.9)
  Top 0.508: v82.7,17.2 83.9,18.4 83.9,31.9 82.15,33.65 73.21,33.65 70.25,30.68 67.78,30.68 65.09,27.99 v54.43,27.99
  Bottom 0.508: U$5.12V 51.82,19.55 U$25.12V_OUT 51.82,26.94 52.87,27.99 v54.43,27.99 | U$6.L2 82.64,17.14 v82.7,17.2
N$14
  Bottom 0.508: U$7.L4 38.15,6.99 37.46,6.3 37.46,4.27 40.13,1.6 48.8,1.6 50.99,3.79 50.99,11.87 53.01,13.89 57.69,13.89 60.4,16.6 65.8,16.6 68.3,14.1 76.97,14.1 U$6.U1
N$15  (via drill 0.9)
  Top 0.508: v45.87,11.06 46.31,11.5 49.56,11.5 49.56,24.41 51.67,26.52 55.04,26.52 55.74,27.23 65.41,27.23 68.1,29.92 70.62,29.92 73.04,32.34 78.1,32.34 79.7,30.73 v79.7,27.63
  Bottom 0.508: v79.7,27.63 82.97,27.63 83.9,26.7 83.9,22.8 83.33,22.23 U$6.L4 | U$7.U2 42.55,11.56 43.04,11.06 v45.87,11.06
N$16  (via drill 0.9)
  Top 0.508: v45.71,16.37 45.71,18.97 45.82,19.08 45.82,24.96 44.4,26.38 | 44.4,26.38 42.08,28.7 36.87,28.7 31.03,34.55 31.03,38.67 32.14,39.79 36.59,39.79 v36.6,39.8 45.8,49 45.8,54.2 47.4,55.8 47.7,55.8 v47.61,55.89 | v45.61,27.59 44.4,26.38 | v69.6,27.1 72.3,24.4 v72.3,16.4 | v40.71,20.33 39.48,21.57 34.58,21.55 32.94,19.9 32.95,17.77 v32.8,17.62
  Bottom 0.508: U$1.5V_2 12.7,62.61 12.7,61.05 15.11,58.65 U$10.5V 16.84,56.39 15.37,54.92 15.37,41.86 16.23,41 33.1,41 35.5,38.6 | 35.5,38.6 36.64,37.46 U$23.5V | U$34.U1 28.84,16.41 31.59,16.41 v32.8,17.62 | v36.6,39.8 35.5,38.7 35.5,38.6 | v40.71,20.33 44.67,16.37 v45.71,16.37 44.56,16.37 43.18,14.99 42.93,14.99 U$7.U1 | v45.61,27.59 45.61,29.19 46.98,30.56 57.65,30.56 63.67,24.54 U$25.SIG U$25.DO 69.62,27.08 v69.6,27.1 | v72.3,16.4 75.9,16.4 76.64,17.14 U$6.U2 | U$41.B2 68.91,35.09 67.51,36.49 67.51,39.55 64.06,43 57.51,43 55.21,45.3 55.21,47.49 52.18,50.52 48.48,50.52 47.5,51.5 47.5,55.79 v47.61,55.89 | 50.69,55.89 50.8,56 U$39.B2 U$40.B2
  Bottom 1.508: U$1.5V_1 U$1.5V_2 | v47.61,55.89 50.69,55.89
N$17
  Bottom 0.508: U$7.U3 42.55,9.02 42.88,8.68 49.18,8.68 50.27,9.77 50.27,12.16 52.73,14.61 57.41,14.61 59.53,16.74 U$5.NMEA
N$19
  Bottom 0.508: U$1.22 35.4,60.8 36.44,59.76 41.12,59.76 43.28,57.59 43.28,54.15 42.45,53.31 19.71,53.31 16.8,50.4 16.8,43.45 U$10.9
N$20
  Bottom 0.508: U$1.24 38,62.71 38,61.1 38.63,60.47 41.41,60.47 43.99,57.89 43.99,53.85 42.74,52.6 21.7,52.6 19.38,50.28 U$10.10
N$21
  Bottom 0.508: U$8.IN_CAP 3.93,54.56 4.87,55.5 8.77,55.5 U$8.IN_V 14.02,55.58 14.66,54.94 14.66,45.47 | U$9.IN_CAP U$9.IN_V 14.61,45.42 14.66,45.47 | U$25.12V_IN 53.57,31.39 53.57,31.35 44.27,31.35 35.79,31.35 34.98,32.16 34.98,38.04 32.79,40.23 15.91,40.23 14.66,41.49 14.66,45.47 | U$23.12V
  Bottom 1.5: U$23.12V 44.27,31.35
N$22
  Bottom 0.508: U$1.26 40.48,62.42 44.71,58.19 44.71,53.55 43.04,51.89 24.29,51.89 21.9,49.5 21.92,49.48 U$10.11
N$23
  Bottom 0.508: U$9.OUT_V U$9.OUT_CAP 5.17,40.13 5.17,38.88 | U$29.PIN 3.5,36.86 3.5,37.21
  Bottom 2: 3.5,37.21 5.17,38.88
N$24  (via drill 0.9)
  Top 0.508: v48.4,41.2 48.08,40.88 47.36,40.88 43.56,37.08 33.72,37.08 v33.5,37.3
  Bottom 0.508: v33.5,37.3 33.5,37.37 31.4,39.47 15.6,39.47 14.93,40.14 12.72,40.14 11.2,38.62 7.63,38.62 6.86,37.85 6.86,36.09 4.74,33.98 U$2.B2 | U$14.B2 50.67,41.2 v48.4,41.2
N$25  (via drill 0.9)
  Top 0.508: v72.21,29.5 72.21,25.57 75.82,21.96 75.82,13.92 76.79,12.95 78.95,12.95 v80,11.9
  Bottom 0.508: U$10.13 40.62,43.41 45.11,47.9 U$14.B1 53.8,47.9 54.5,47.2 54.5,45 57.27,42.23 63.75,42.23 66.8,39.18 66.8,34.5 67.65,33.65 70.22,33.65 72.21,31.66 v72.21,29.5 | U$6.L1 v80.01,11.91 v80,11.9
N$26
  Bottom 0.508: U$31.PIN 42.93,22.43 42.5,22 36.06,22 35.5,21.44 22.66,21.44 21.11,22.99 21.11,28.75 19.32,30.54 9.06,30.54 7.28,32.32 U$2.B1
N$27  (via drill 0.9)
  Top 0.508: v34.9,45.8 34.9,44.56 29.6,39.26 29.6,33.8 33.1,30.3 33.1,28.5 v30.8,26.2
  Bottom 0.508: U$33.PIN 33.23,28.27 32.1,29.4 U$15.B2 30.8,29.03 v30.8,26.2 | U$17.B2 36.45,47.35 v34.9,45.8
N$28
  Bottom 0.508: U$3.B2 12.64,32.06 13.37,31.33 19.8,31.33 21.73,29.4 U$15.B1
N$29  (via drill 0.9, 0.9 pad 1.3)
  Top 0.508: v24.07,42.45 24.07,42.34 22.72,41 17.42,41 13.34,36.91 v12.79,36.91 | v16.5,36.7 16.5,38.98 17.79,40.27 25.8,40.27 26.75,39.33 v26.75,35.7 | v27.59,30.41 27.46,30.41 24.87,27.81 22.48,27.81 21.1,26.44 21.1,5.51 24.12,2.49 27.99,2.49 28.7,3.2 28.69,3.21 28.69,4.1 29.38,4.79 30.21,4.79 30.22,4.8 30.6,4.8 31.37,4.03 35.32,4.03 36.3,5 36.3,7.79 v37.52,9.01
  Bottom 0.508: U$16.B1 25,48.7 23.5,47.2 23.5,43.02 v24.07,42.45 | v12.79,36.91 12.89,36.91 15.18,34.62 U$3.B1 15.18,35.38 v16.5,36.7 | v26.75,35.7 26.73,35.68 26.73,31.93 27.59,31.07 v27.59,30.41 | v37.52,9.01 37.39,9.14 37.78,9.53 U$7.L3
N$30  (via drill 0.9)
  Top 0.508: v43.55,29.38 44.57,29.38 45.79,30.6 62,30.6 v62.6,30
  Bottom 0.508: U$4.B1 23.1,35.4 24.2,36.5 24.2,38.2 24.71,38.71 31.08,38.71 32.03,37.76 32.03,36.69 32.89,35.83 33.79,35.83 34.22,35.4 34.22,31.84 36.69,29.38 v43.55,29.38 | v62.6,30 64.88,30 U$25.GND U$25.DI
N$31  (via drill 0.9)
  Top 0.508: v24.99,46.61 25.52,46.08 25.52,41.57 28.18,38.91 28.18,35.12 27.34,34.28 25.51,34.28 22.85,36.94 v22.25,36.94
  Bottom 0.508: U$18.B1 41.81,45.61 40.33,44.13 29.3,44.13 27.61,45.82 25.78,45.82 v24.99,46.61 | U$4.B2 20.56,35.27 22.24,36.95 v22.25,36.94
N$32
  Bottom 0.508: U$1.38 55.81,62.67 55.81,60.45 59.57,56.7 65.25,56.7 68.89,60.34 74.52,60.34 82.97,51.88 82.97,33.4 78.27,28.7 78.27,25.57 U$6.U5
N$33
  Bottom 0.508: U$1.12 22.7,61.25 24.9,59.05 40.75,59.05 41.81,57.99 U$18.B2
N$34
  Bottom 0.508: U$1.36 52.97,62.77 52.95,62.79 52.95,61.81 58.79,55.98 65.55,55.98 69.15,59.57 74.25,59.57 82.24,51.59 82.24,33.69 77.56,29.01 77.56,27.19 75.82,25.45 75.82,23.88 U$6.U4
N$35  (via drill 0.9)
  Top 0.508: v35.2,2.6 43.52,2.6 v45.06,4.15
  Bottom 0.508: U$34.L2 22.16,12.06 21.11,11.01 21.11,5.55 25.56,1.1 33.7,1.1 v35.2,2.6 | U$7.U5 44.76,4.45 v45.06,4.15
N$36
  Bottom 0.508: U$34.U2 27.11,12 29.93,12 34.47,7.46 U$35.B2
N$37  (via drill 0.9)
  Top 0.508: v72.82,43.59 72.82,47.32 65.74,54.4 59.8,54.4 53.08,61.12 48.32,61.12 47.72,60.52 v29.27,60.52
  Bottom 0.508: U$1.16 27.77,61.92 29.18,60.52 v29.27,60.52 | U$38.PIN 72.82,40.12 v72.82,43.59
N$38
  Bottom 0.508: U$34.L5 24.5,3.3 25.95,1.85 31.35,1.85 32.1,2.6 U$37.B2
N$39  (via drill 0.9)
  Top 0.508: v22.55,8.24 22.8,8.49 22.8,16.3 v25.3,18.8
  Bottom 0.508: U$34.L4 23.8,6.99 v22.55,8.24 | v25.3,18.8 26.3,19.8 U$36.B2
N$40
  Bottom 0.508: U$7.L1 40.01,16.39 36.83,19.57 U$36.B1
N$42  (via drill 0.9)
  Top 0.508: v82.4,30.8 v82.4,24.8
  Bottom 0.508: U$1.40 58.26,59.02 59.87,57.41 64.95,57.41 68.64,61.1 74.76,61.1 83.7,52.16 83.7,31.2 83.3,30.8 v82.4,30.8 | U$6.L5 82.36,24.77 v82.4,24.8

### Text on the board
tPlace: GND | 5V | 10uF | 5V | ETH. / JACK | 3.3V / REG. | GND | 10Kohm | 330ohm | 1.5Kohm | 2.2Kohm | 22uF | FUSE | 330nF | 33Kohm | GND | INPUT / LED + | 9V LDO / REG. | GND | 22uF | To PWR / Switch | INPUT / SIGNAL | 5V IN | 12V IN | 680ohm | CAM / 9V / PWR | BATT | GND | GND | To 12 and 5 / Volt Reg. | GND | NPN | NPN | NPN | BATT / IN | 330ohm | RELAY | GND | GND | GND | 3.3V | APX18 / PCB | 1N4001 / <--DIODE-- | CAM. / FEED- / BACK | 3.3V / CAM / LEMO | NAV / Switch | 3.3V | CAM. / TRIG. | COM3 / TX n/c | 2.2Kohm | TD- | TD+ | RD- | RD+ | 12V | GND | PPS | NMEA | LIDAR SENSOR | 680ohm | 680ohm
